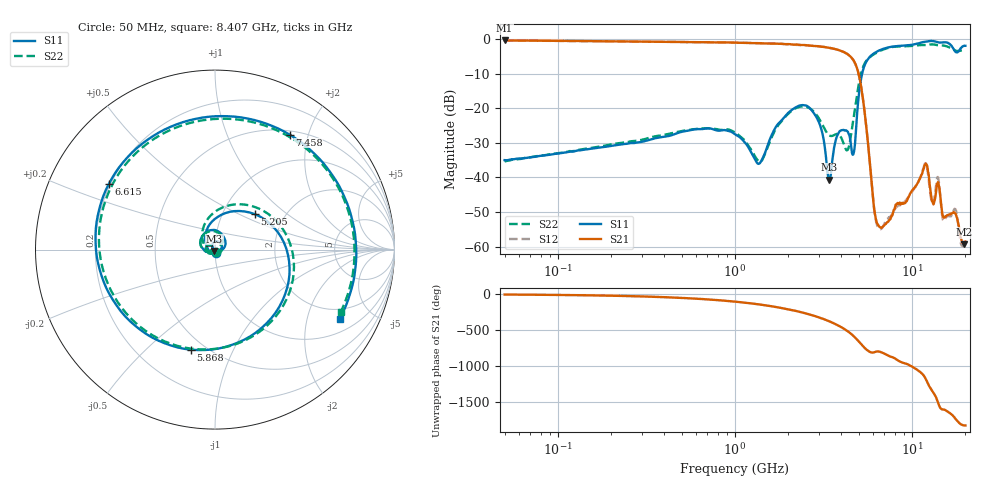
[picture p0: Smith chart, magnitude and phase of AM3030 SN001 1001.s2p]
# Hz S DB R 50
!freq MagS11 AngS11 MagS21 AngS21 MagS12 AngS12 MagS22 AngS22
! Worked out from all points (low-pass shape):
!   1601 points, 50 MHz to 20.05 GHz, reference 50 ohm
!   highest |S21| = -0.40 dB at 50 MHz (marker M1); lowest = -59.3 dB at 19.6 GHz (marker M2)
!   |S21| within 3 dB of the highest: start of sweep to 3.969 GHz
!   lowest |S11| = -40.7 dB at 3.408 GHz (marker M3), VSWR 1.02, Z = 49.5 - j0.802 ohm
!   |S11| at or under -10 dB: start of sweep to 5.232 GHz
!   |S22| runs from -35.4 to -1.5 dB; largest |S21 - S12| = 0.013
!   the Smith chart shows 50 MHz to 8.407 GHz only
!   S11 on the Smith chart (normalised r, x): 50 MHz: 1.01, -0.03; 5.205 GHz: 1.42, +0.61; 5.868 GHz: 0.42, -0.70; 6.615 GHz: 0.19, +0.27; 7.458 GHz: 0.55, +1.70; 8.407 GHz: 1.52, -3.18
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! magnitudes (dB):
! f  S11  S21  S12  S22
! 50 MHz  -35.0  -0.4  -0.4  -35.4
! 135.9 MHz  -32.1  -0.6  -0.6  -31.9
! 369.6 MHz  -28.5  -0.8  -0.8  -28.0
! 1.005 GHz  -27.6  -1.1  -1.0  -27.0
! 1.366 GHz  -36.1  -1.2  -1.2  -35.4
! 1.995 GHz  -21.4  -1.5  -1.5  -21.7
! 2.722 GHz  -20.7  -1.9  -1.9  -20.5
! 3.408 GHz  -40.7  -2.5  -2.5  -27.8
! 3.814 GHz  -27.6  -3.1  -3.1  -27.5
! 4.348 GHz  -26.8  -4.4  -4.4  -31.9
! 4.687 GHz  -33.0  -6.2  -6.2  -22.5
! 5.205 GHz  -10.5  -14.8  -14.8  -9.2
! 5.868 GHz  -4.8  -39.2  -39.1  -5.0
! 6.615 GHz  -3.2  -54.4  -54.9  -3.4
! 7.402 GHz  -2.4  -52.5  -51.7  -2.5
! 7.458 GHz  -2.3  -52.3  -51.5  -2.5
! 8.407 GHz  -2.0  -47.6  -48.1  -2.1
! 11.91 GHz  -0.8  -36.2  -35.9  -1.7
! 12.98 GHz  -0.5  -46.9  -47.4  -1.5
! 13.99 GHz  -0.9  -41.4  -39.8  -1.8
! 19.6 GHz  -2.0  -59.3  -59.2  -3.2
! 20.05 GHz  -1.9  -58.5  -58.3  -3.2
